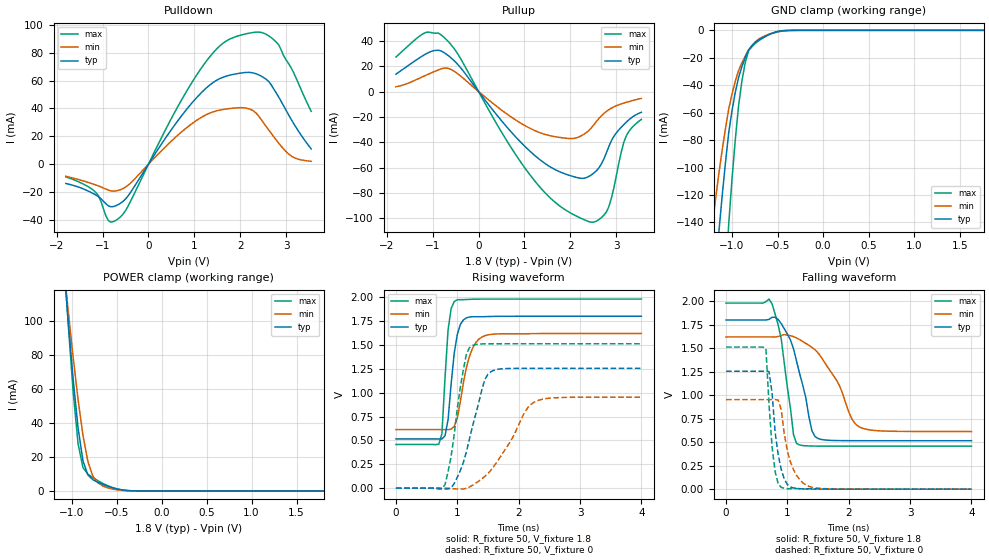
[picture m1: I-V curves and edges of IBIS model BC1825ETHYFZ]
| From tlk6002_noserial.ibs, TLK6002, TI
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[Model]   BC1825ETHYFZ
Model_type   I/O
Polarity   Non-Inverting
Enable   Active-Low
Vinl =  0.63
Vinh =  1.17
Cref =  15.0000pF
Rref =  100.0000M
Vref =  0V
Vmeas =  0.9
C_comp   1.756427p   1.323266p   2.339455p
[Model Spec]
Vinl   0.63   0.567   0.693
Vinh   1.17   1.053   1.287
[Temperature Range]   25   125   -40
[Voltage Range]   1.8   1.62   1.98
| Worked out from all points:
|   slope of the pulldown table from 0 to 0.27 V, typ, clamps not added: 19.6 ohm
|   slope of the pullup table from 0 to 0.27 V, typ, clamps not added: 21.2 ohm
|   GND clamp passes 1 mA (typ) near -0.50 V on its own axis
|   POWER clamp passes 1 mA (typ) near -0.48 V on its own axis
|   rising waveform, R_fixture 50, V_fixture 1.8: 20-80 % time 126ps typ, 198ps min, 87.5ps max; typ from 0.516 V to 1.8 V
|   rising waveform, R_fixture 50, V_fixture 0: 20-80 % time 302ps typ, 522ps min, 201ps max; typ from 0 V to 1.25 V
|   falling waveform, R_fixture 50, V_fixture 1.8: 20-80 % time 277ps typ, 470ps min, 194ps max; typ from 1.8 V to 0.516 V
|   falling waveform, R_fixture 50, V_fixture 0: 20-80 % time 134ps typ, 197ps min, 104ps max; typ from 1.25 V to 0 V
[POWER_clamp]
-1.8V     671.8mA    545.1mA    808.2mA
-1.073V   123.7mA    124.6mA    127.1mA
-1.055V   111.5mA    115mA      112.4mA
-981.8mV  65.6mA     78.46mA    58.15mA
-927.3mV  37.01mA    53.65mA    27.72mA
-872.7mV  17.65mA    32.56mA    13.64mA
-818.2mV  9.375mA    17.27mA    9.824mA
-763.6mV  6.606mA    8.774mA    7.806mA
-654.5mV  3.864mA    2.942mA    4.49mA
-490.9mV  1.152mA    622.6uA    1.11mA
-327.3mV  85.89uA    40.76uA    54.47uA
1.8V      224.8nA    189.7nA    319.8nA
[Pulldown]
-1.8V     -13.79mA   -8.604mA   -9.047mA
-1.145V   -22.07mA   -14.92mA   -20.24mA
-872.7mV  -29.86mA   -18.56mA   -40.41mA
-654.5mV  -28.9mA    -18.77mA   -39.05mA
-436.4mV  -22.41mA   -14.91mA   -29.64mA
1.091V    49.25mA    32.39mA    66.03mA
1.582V    61.86mA    39.02mA    85.71mA
2.018V    65.47mA    40.6mA     92.73mA
2.345V    64.89mA    36.67mA    94.82mA
2.782V    51.24mA    17.42mA    87.77mA
3.109V    32.2mA     5.915mA    69.14mA
3.545V    10.99mA    2.102mA    37.97mA
[Pullup]
-1.8V     13.68mA    3.76mA     27.17mA
-1.145V   29.68mA    12.85mA    46.61mA
-763.6mV  30.98mA    18.39mA    43.09mA
-436.4mV  20.7mA     13.56mA    28.7mA
545.5mV   -25mA      -15.84mA   -34.72mA
1.2V      -49.7mA    -30.43mA   -69.45mA
2.018V    -66.57mA   -37.11mA   -96.11mA
2.4V      -67.01mA   -30.75mA   -102.6mA
2.782V    -48.63mA   -15.78mA   -95.19mA
2.891V    -38.89mA   -13.16mA   -84.37mA
3.164V    -26.08mA   -9.131mA   -40.05mA
3.545V    -16.39mA   -5.461mA   -21.97mA
[GND_clamp]
-1.8V     -733.8mA   -497.1mA   -1.291A
-1.218V   -206.8mA   -143.2mA   -384.4mA
-1.145V   -148mA     -104.9mA   -278.9mA
-1.109V   -121.5mA   -87.8mA    -229.9mA
-1.036V   -74.74mA   -57.48mA   -141.5mA
-963.6mV  -45.13mA   -37mA      -79.59mA
-927.3mV  -34.3mA    -29.23mA   -54.66mA
-890.9mV  -26.43mA   -23.61mA   -36.81mA
-818.2mV  -14.35mA   -14.32mA   -14.96mA
-709.1mV  -6.982mA   -6.478mA   -7.736mA
-418.2mV  -220.1uA   -368.1uA   -103.1uA
1.764V    204.4nA    959.6nA    204.4nA
[Ramp]
dV/dt_f  0.7911936/0.2872552n  0.6188735/0.488238n   0.9397716/0.2004116n
dV/dt_r  0.7583382/0.3036187n  0.5768991/0.5283491n  0.9134414/0.2030853n
R_load = 50
[Rising Waveform]
R_fixture = 50
V_fixture = 1.8
V_fixture_min = 1.62
V_fixture_max = 1.98
0s        515.6mV    613.4mV    457.9mV
700ps     515.4mV    613.4mV    461.2mV
750ps     515.1mV    613.5mV    571.5mV
800ps     548.3mV    613.7mV    1.155V
850ps     717.4mV    612.7mV    1.659V
900ps     1.093V     618.5mV    1.881V
1ns       1.609V     733.8mV    1.973V
1.2ns     1.792V     1.383V     1.977V
1.4ns     1.795V     1.582V     1.98V
4ns       1.8V       1.62V      1.98V
[Rising Waveform]
R_fixture = 50
V_fixture = 0
V_fixture_min = 0
V_fixture_max = 0
0s        770.2nV    748.4nV    867.8nV
800ps     -9.101mV   337.4uV    36.46mV
950ps     49.28mV    -7.17mV    563.1mV
1.05ns    184.9mV    -8.299mV   1.058V
1.15ns    385.1mV    -1.425mV   1.407V
1.25ns    651.6mV    31.2mV     1.495V
1.4ns     1.03V      97.98mV    1.51V
1.5ns     1.193V     153.4mV    1.512V
2.25ns    1.255V     899.5mV    1.512V
4ns       1.255V     952.8mV    1.512V
[Falling Waveform]
R_fixture = 50
V_fixture = 1.8
V_fixture_min = 1.62
V_fixture_max = 1.98
0s        1.8V       1.62V      1.98V
750ps     1.829V     1.62V      1.972V
900ps     1.761V     1.635V     1.596V
1.1ns     1.492V     1.623V     577.9mV
1.15ns    1.36V      1.609V     486.6mV
1.4ns     620.2mV    1.509V     458.9mV
1.5ns     538.6mV    1.449V     458.2mV
2.05ns    515.9mV    747.8mV    457.9mV
2.2ns     515.7mV    653.5mV    457.9mV
4ns       515.6mV    613.4mV    457.9mV
[Falling Waveform]
R_fixture = 50
V_fixture = 0
V_fixture_min = 0
V_fixture_max = 0
0s        1.255V     952.8mV    1.512V
650ps     1.255V     952.8mV    1.493V
700ps     1.252V     952.8mV    905.1mV
750ps     1.025V     952.7mV    450.9mV
800ps     607.6mV    954.1mV    185.8mV
900ps     209.2mV    844.8mV    18.9mV
950ps     105.4mV    583.9mV    9.035mV
1.05ns    23.66mV    287.8mV    4.752mV
1.35ns    5.405mV    30.23mV    1.017mV
4ns       770.2nV    1.66uV     867.8nV
